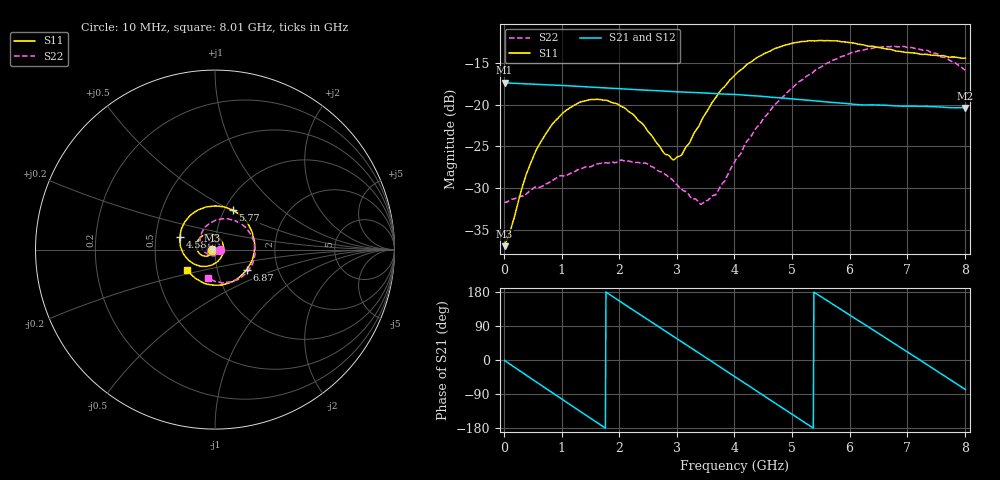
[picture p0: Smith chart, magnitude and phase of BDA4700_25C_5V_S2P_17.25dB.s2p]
!Agilent Technologies,E5071B,MY42404982,A.09.10
!Date: Mon Oct 20 13:34:55 2025
!Data & Calibration Information:
!Freq	S11:SOLT2(ON)	S21:SOLT2(ON)	S12:SOLT2(ON)	S22:SOLT2(ON)
# Hz S RI R 50
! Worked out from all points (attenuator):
!   801 points, 10 MHz to 8.01 GHz, reference 50 ohm
!   highest |S21| = -17.35 dB at 10 MHz (marker M1); lowest = -20.4 dB at 8.01 GHz (marker M2)
!   lowest |S11| = -37.0 dB at 10 MHz (marker M3), VSWR 1.03, Z = 48.6 - j0.142 ohm
!   |S11| at or under -10 dB: start of sweep to end of sweep
!   |S22| runs from -31.9 to -13.0 dB; largest |S21 - S12| = 0.0011
!   S11 on the Smith chart (normalised r, x): 10 MHz: 0.97, -0.00; 4.58 GHz: 0.67, +0.10; 5.77 GHz: 1.09, +0.51; 6.87 GHz: 1.38, -0.32; 8.01 GHz: 0.72, -0.17
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1e7  -0.0141 -0.00147  0.1357 -0.00295  0.1357 -0.00307  0.026 -0.000883
1.2e8  -0.0154 -0.00921  0.1314 -0.0298  0.1314 -0.0298  0.0263 -0.00575
3.7e8  -0.0254 -0.0265  0.1047 -0.0831  0.1046 -0.0832  0.0216 -0.0191
5.8e8  -0.042 -0.0358  0.0664 -0.1148  0.0663 -0.1149  0.0138 -0.029
8.8e8  -0.0726 -0.0321  -0.00131 -0.1311  -0.00141 -0.1313  -0.00758 -0.035
1.35e9  -0.1035 0.0147  -0.0961 -0.0856  -0.0962 -0.0856  -0.0378 -0.0169
2.07e9  -0.0403 0.0877  -0.1069 0.0641  -0.1069 0.0642  -0.0287 0.0362
2.68e9  0.0404 0.0408  0.00393 0.1213  0.00394 0.1212  0.017 0.0363
2.97e9  0.046 -0.0108  0.0611 0.103  0.0611 0.1029  0.0284 0.0182
3.1e9  0.0384 -0.0336  0.0824 0.0862  0.0822 0.0865  0.0299 0.00735
3.43e9  -0.00685 -0.0804  0.1146 0.0277  0.1147 0.0277  0.0181 -0.0176
3.69e9  -0.0616 -0.0933  0.1139 -0.0247  0.114 -0.025  -0.00226 -0.0291
4.01e9  -0.1339 -0.0689  0.0826 -0.0804  0.0827 -0.0803  -0.0364 -0.0274
4.58e9  -0.1956 0.0682  -0.0219 -0.1093  -0.0218 -0.1095  -0.0816 0.0346
4.92e9  -0.1599 0.1649  -0.0774 -0.077  -0.0773 -0.0773  -0.0744 0.0927
5.35e9  -0.0434 0.2383  -0.1059 -0.00407  -0.1059 -0.00438  -0.0137 0.1542
5.77e9  0.0986 0.2211  -0.0799 0.0647  -0.0797 0.0648  0.083 0.1689
6.23e9  0.2042 0.1033  -0.0115 0.099  -0.0106 0.0992  0.1837 0.107
6.68e9  0.2091 -0.053  0.0601 0.0786  0.0603 0.0786  0.2228 -0.00858
6.87e9  0.1766 -0.1121  0.0813 0.0553  0.0815 0.0548  0.2142 -0.0629
7.43e9  0.00907 -0.1982  0.0911 -0.0345  0.0912 -0.0348  0.1104 -0.1718
8.01e9  -0.1536 -0.1128  0.02 -0.0937  0.0202 -0.0938  -0.0386 -0.1562
